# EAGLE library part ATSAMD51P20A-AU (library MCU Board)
SAMD51 Series 1 MB Flash 256 kB RAM 32-Bit SMT Microcontroller - TQFP-128
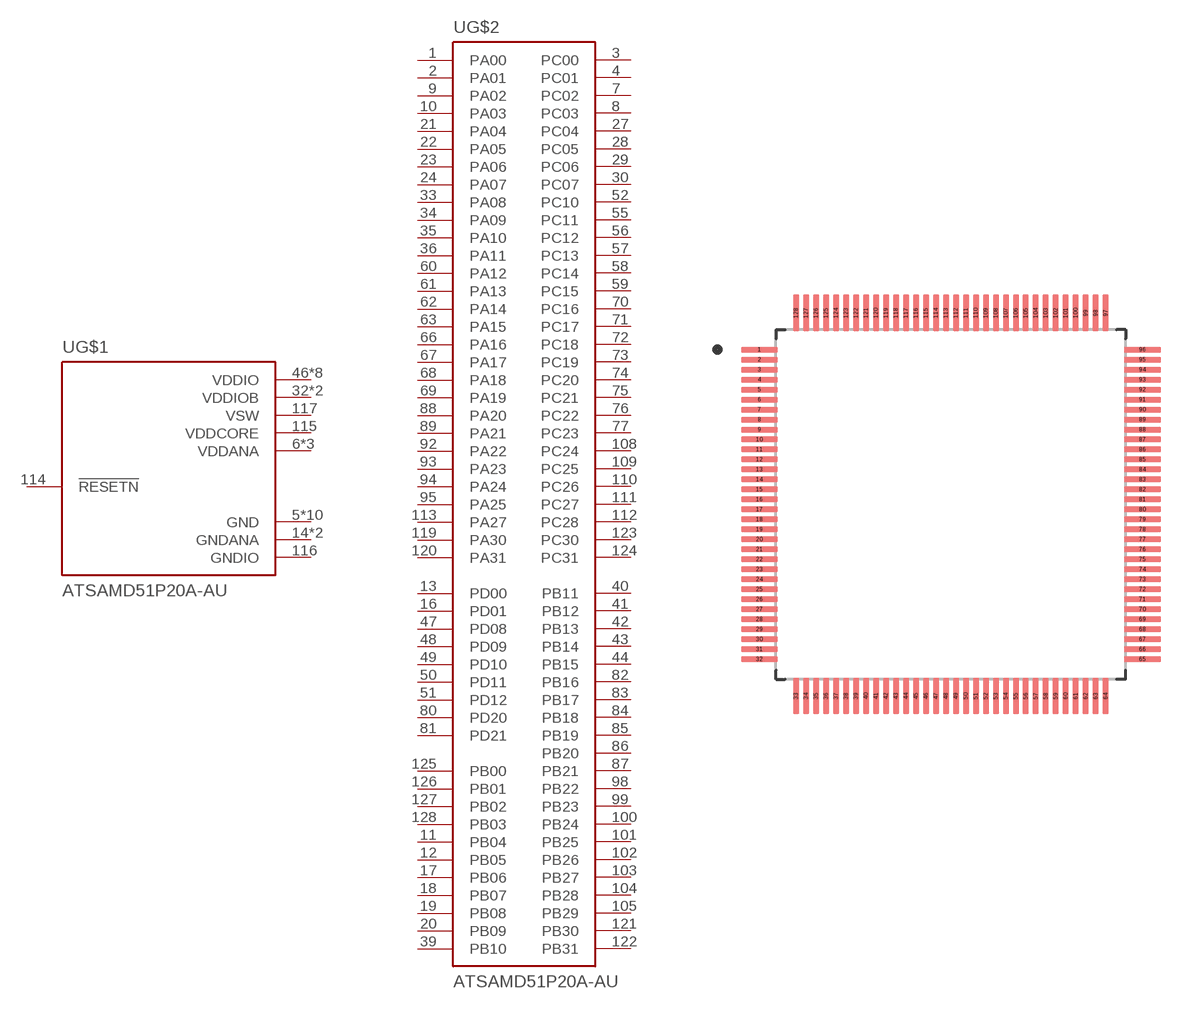
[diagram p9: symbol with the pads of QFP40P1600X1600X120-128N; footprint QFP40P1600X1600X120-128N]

Designator prefix U; gates G$1=ATSAMD51P20A-AU_SECTION1 G$2=ATSAMD51P20A-AU_SECTION2

## ATSAMD51P20A-AU (AVAILABILITY: Unavailable; DESCRIPTION: ARM® Cortex®-M4F SAM D51 Microcontroller IC 32-Bit 120MHz 1MB (1M x 8) FLASH 128-TQFP (14x14); MF: Microchip; MP: ATSAMD51P20A-AU; PACKAGE: TQFP-128 Microchip; PRICE: None)  [QFP40P1600X1600X120-128N]
1  G$2:PA00
2  G$2:PA01
3  G$2:PC00
4  G$2:PC01
5  G$1:GND  pwr
6  G$1:VDDANA  pwr
7  G$2:PC02
8  G$2:PC03
9  G$2:PA02
10  G$2:PA03
11  G$2:PB04
12  G$2:PB05
13  G$2:PD00
14  G$1:GNDANA  pwr
15  G$1:VDDANA  pwr
16  G$2:PD01
17  G$2:PB06
18  G$2:PB07
19  G$2:PB08
20  G$2:PB09
21  G$2:PA04
22  G$2:PA05
23  G$2:PA06
24  G$2:PA07
25  G$1:GNDANA  pwr
26  G$1:VDDANA  pwr
27  G$2:PC04
28  G$2:PC05
29  G$2:PC06
30  G$2:PC07
31  G$1:GND  pwr
32  G$1:VDDIOB  pwr
33  G$2:PA08
34  G$2:PA09
35  G$2:PA10
36  G$2:PA11
37  G$1:VDDIOB  pwr
38  G$1:GND  pwr
39  G$2:PB10
40  G$2:PB11
41  G$2:PB12
42  G$2:PB13
43  G$2:PB14
44  G$2:PB15
45  G$1:GND  pwr
46  G$1:VDDIO  pwr
47  G$2:PD08
48  G$2:PD09
49  G$2:PD10
50  G$2:PD11
51  G$2:PD12
52  G$2:PC10
53  G$1:GND  pwr
54  G$1:VDDIO  pwr
55  G$2:PC11
56  G$2:PC12
57  G$2:PC13
58  G$2:PC14
59  G$2:PC15
60  G$2:PA12
61  G$2:PA13
62  G$2:PA14
63  G$2:PA15
64  G$1:GND  pwr
65  G$1:VDDIO  pwr
66  G$2:PA16
67  G$2:PA17
68  G$2:PA18
69  G$2:PA19
70  G$2:PC16
71  G$2:PC17
72  G$2:PC18
73  G$2:PC19
74  G$2:PC20
75  G$2:PC21
76  G$2:PC22
77  G$2:PC23
78  G$1:GND  pwr
79  G$1:VDDIO  pwr
80  G$2:PD20
81  G$2:PD21
82  G$2:PB16
83  G$2:PB17
84  G$2:PB18
85  G$2:PB19
86  G$2:PB20
87  G$2:PB21
88  G$2:PA20
89  G$2:PA21
90  G$1:GND  pwr
91  G$1:VDDIO  pwr
92  G$2:PA22
93  G$2:PA23
94  G$2:PA24
95  G$2:PA25
96  G$1:GND  pwr
97  G$1:VDDIO  pwr
98  G$2:PB22
99  G$2:PB23
100  G$2:PB24
101  G$2:PB25
102  G$2:PB26
103  G$2:PB27
104  G$2:PB28
105  G$2:PB29
106  G$1:GND  pwr
107  G$1:VDDIO  pwr
108  G$2:PC24
109  G$2:PC25
110  G$2:PC26
111  G$2:PC27
112  G$2:PC28
113  G$2:PA27
114  G$1:!RESETN  in
115  G$1:VDDCORE  pwr
116  G$1:GNDIO  pwr
117  G$1:VSW  pwr
118  G$1:VDDIO  pwr
119  G$2:PA30
120  G$2:PA31
121  G$2:PB30
122  G$2:PB31
123  G$2:PC30
124  G$2:PC31
125  G$2:PB00
126  G$2:PB01  out
127  G$2:PB02  out
128  G$2:PB03

## Footprint QFP40P1600X1600X120-128N (pad centres in mm)
smd 1.47 x 0.24: 1 -7.67,6.2; 2 -7.67,5.8; 3 -7.67,5.4; 4 -7.67,5; 5 -7.67,4.6; 6 -7.67,4.2; 7 -7.67,3.8; 8 -7.67,3.4; 9 -7.67,3; 10 -7.67,2.6; 11 -7.67,2.2; 12 -7.67,1.8; 13 -7.67,1.4; 14 -7.67,1; 15 -7.67,0.6; 16 -7.67,0.2; 17 -7.67,-0.2; 18 -7.67,-0.6; 19 -7.67,-1; 20 -7.67,-1.4; 21 -7.67,-1.8; 22 -7.67,-2.2; 23 -7.67,-2.6; 24 -7.67,-3; 25 -7.67,-3.4; 26 -7.67,-3.8; 27 -7.67,-4.2; 28 -7.67,-4.6; 29 -7.67,-5; 30 -7.67,-5.4; 31 -7.67,-5.8; 32 -7.67,-6.2; 65 7.67,-6.2; 66 7.67,-5.8; 67 7.67,-5.4; 68 7.67,-5; 69 7.67,-4.6; 70 7.67,-4.2; 71 7.67,-3.8; 72 7.67,-3.4; 73 7.67,-3; 74 7.67,-2.6; 75 7.67,-2.2; 76 7.67,-1.8; 77 7.67,-1.4; 78 7.67,-1; 79 7.67,-0.6; 80 7.67,-0.2; 81 7.67,0.2; 82 7.67,0.6; 83 7.67,1; 84 7.67,1.4; 85 7.67,1.8; 86 7.67,2.2; 87 7.67,2.6; 88 7.67,3; 89 7.67,3.4; 90 7.67,3.8; 91 7.67,4.2; 92 7.67,4.6; 93 7.67,5; 94 7.67,5.4; 95 7.67,5.8; 96 7.67,6.2
smd 0.24 x 1.47: 33 -6.2,-7.67; 34 -5.8,-7.67; 35 -5.4,-7.67; 36 -5,-7.67; 37 -4.6,-7.67; 38 -4.2,-7.67; 39 -3.8,-7.67; 40 -3.4,-7.67; 41 -3,-7.67; 42 -2.6,-7.67; 43 -2.2,-7.67; 44 -1.8,-7.67; 45 -1.4,-7.67; 46 -1,-7.67; 47 -0.6,-7.67; 48 -0.2,-7.67; 49 0.2,-7.67; 50 0.6,-7.67; 51 1,-7.67; 52 1.4,-7.67; 53 1.8,-7.67; 54 2.2,-7.67; 55 2.6,-7.67; 56 3,-7.67; 57 3.4,-7.67; 58 3.8,-7.67; 59 4.2,-7.67; 60 4.6,-7.67; 61 5,-7.67; 62 5.4,-7.67; 63 5.8,-7.67; 64 6.2,-7.67; 97 6.2,7.67; 98 5.8,7.67; 99 5.4,7.67; 100 5,7.67; 101 4.6,7.67; 102 4.2,7.67; 103 3.8,7.67; 104 3.4,7.67; 105 3,7.67; 106 2.6,7.67; 107 2.2,7.67; 108 1.8,7.67; 109 1.4,7.67; 110 1,7.67; 111 0.6,7.67; 112 0.2,7.67; 113 -0.2,7.67; 114 -0.6,7.67; 115 -1,7.67; 116 -1.4,7.67; 117 -1.8,7.67; 118 -2.2,7.67; 119 -2.6,7.67; 120 -3,7.67; 121 -3.4,7.67; 122 -3.8,7.67; 123 -4.2,7.67; 124 -4.6,7.67; 125 -5,7.67; 126 -5.4,7.67; 127 -5.8,7.67; 128 -6.2,7.67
